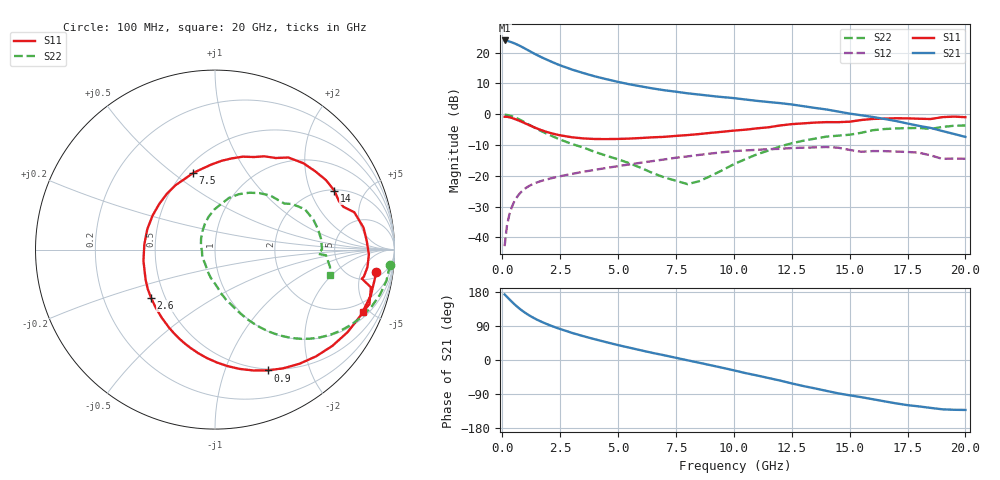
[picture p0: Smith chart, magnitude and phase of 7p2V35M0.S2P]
! Infineon Technologies  Discrete & RF Semiconductors
! bfp620
! VCE =  2.3 V,  IC =  5.0 mA
! Common Emitter S-Parameters:  Sep 2002
# GHz  S  MA  R  50
!  f  S11  S21  S12  S22
! GHz  MAG  ANG  MAG  ANG  MAG  ANG  MAG  ANG
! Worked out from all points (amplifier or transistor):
!   59 points, 100 MHz to 20 GHz, reference 50 ohm
!   highest |S21| = 23.9 dB at 100 MHz (marker M1)
!   |S21| within 3 dB of that: start of sweep to 1.071 GHz
!   unconditionally stable (mu >= 1): 4.762 GHz to 11.71 GHz; 14.69 GHz to 15.31 GHz; 17.23 GHz to end of sweep
!   at 1 GHz: K = 0.33, MSG = 22.6 dB, |S12| = -24.1 dB
!   at 5.5 GHz: K = 1.05, MAG = 11.7 dB, |S12| = -16.3 dB
!   at 20 GHz: K = 1.31, MAG = 0.2 dB, |S12| = -14.5 dB
!   S11 on the Smith chart (normalised r, x): 100 MHz: 7, -10; 900 MHz: 0.48, -1.41; 2.6 GHz: 0.42, -0.28; 7.5 GHz: 0.56, +0.59; 14 GHz: 2.05, +2.99; 20 GHz: 1.34, -4.58
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0.1  0.9076 -8.0  15.7 173.0  0.0072 69.9  0.9788 -5.1
0.2  0.9052 -16.2  15.48 166.7  0.0153 76.3  0.9709 -10.3
0.3  0.8912 -24.2  15.12 160.5  0.0231 74.5  0.9529 -15.3
0.5  0.8457 -39.4  14.21 148.5  0.0371 67.8  0.8987 -24.7
0.7  0.7909 -53.6  13.15 137.8  0.0488 61.3  0.8324 -32.9
0.9  0.7339 -66.5  12.05 128.4  0.0585 55.6  0.7622 -39.9
1.2  0.6531 -83.8  10.45 116.4  0.0697 48.7  0.6613 -48.3
1.4  0.6062 -94.2  9.518 109.6  0.0755 45.1  0.6019 -52.7
1.6  0.5662 -103.6  8.719 103.5  0.0804 42.2  0.5502 -56.4
2  0.5043 -120.6  7.437 93.0  0.0888 37.8  0.4672 -62.2
2.6  0.4464 -143.0  5.998 79.7  0.1 33.1  0.3741 -69.0
3  0.4216 -156.5  5.306 71.7  0.1071 30.5  0.3284 -72.7
3.5  0.4036 -171.1  4.644 62.9  0.1162 27.5  0.2872 -77.4
5  0.3961 151.4  3.339 39.3  0.1435 18.8  0.1849 -91.1
7  0.4283 113.3  2.443 12.4  0.1841 5.8  0.0939 -127.1
7.5  0.4438 106.0  2.313 5.8  0.1963 1.8  0.0831 -148.4
10.5  0.5595 67.2  1.728 -34.5  0.2578 -26.7  0.1864 101.0
12  0.6556 51.5  1.51 -54.3  0.2736 -41.1  0.2989 74.7
13.5  0.7295 32.1  1.263 -74.9  0.2884 -57.2  0.4007 51.7
14  0.742 26.2  1.191 -81.5  0.2932 -63.5  0.4317 44.2
17  0.8578 -1.9  0.774 -114.4  0.2471 -88.0  0.5855 11.0
20  0.8927 -22.8  0.427 -131.8  0.1886 -102.1  0.6556 -12.3
